FUNCTION "MISCL" : VOID
TITLE =
VERSION : 0.1

BEGIN
NETWORK
TITLE =Nuova gestione blocchi laterali

//Creazione dell'impulso di sblocco fermi laterali non appena inizia
//la fase di fusione definita da M22.4
      U     "CA.AF";
      L     S5T#1S500MS;
      SI    T     57;
      U     T     57;
      U     "E       1.1";
      =     "M40.0";
//Richiusura dei fermi laterali con due secondi di anticipo rispetto
//alla fine del tempo di attesa fusione
      U     "CA.AF";
      L     "T.AF";
      L     10;
      <=I   ;
      L     S5T#1S500MS;
      SI    T     58;
      U     T     58;
      U     "E       1.1";
      =     "M40.1";
END_FUNCTION

